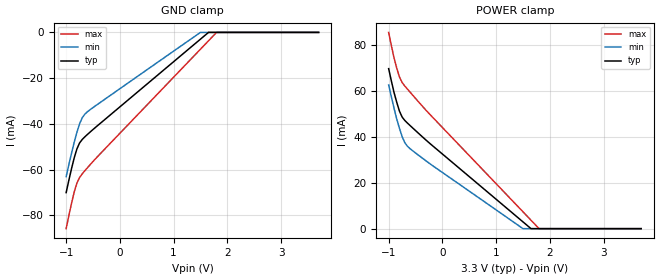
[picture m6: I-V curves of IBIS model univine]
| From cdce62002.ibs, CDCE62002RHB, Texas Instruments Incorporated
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|   Model   univine
[Model]   univine
Model_type   Input
Polarity   Non-Inverting
Vinl   =   1.30
Vinh   =   1.80
|Variable   typ   min   max
C_comp   9.336e-13   4.738e-14   2.334e-12
|Variable   typ   min   max
[Voltage range]   3.3   3.0   3.6
|Variable   typ   min   max
[Temperature range]  25   85   0
[GND_clamp]
|Volts   typ   min   max
-1V       -70.09mA   -63.08mA   -85.83mA
-900mV    -59.59mA   -52.85mA   -74.75mA
-850mV    -54.89mA   -48.07mA   -69.84mA
-800mV    -50.98mA   -43.69mA   -65.93mA
-750mV    -48.35mA   -39.98mA   -63.46mA
-700mV    -46.81mA   -37.31mA   -61.86mA
-650mV    -45.64mA   -35.7mA    -60.45mA
-400mV    -40.48mA   -31.22mA   -53.93mA
1.5V      -2.961mA   0A         -7.354mA
1.65V     0A         0A         -3.677mA
1.8V      0A         0A         0A
3.7V      0A         0A         0A
[POWER_clamp]
|Volts   typ   min   max
-1V       69.73mA    62.62mA    85.53mA
-900mV    59.36mA    52.54mA    74.41mA
-850mV    55.14mA    47.83mA    70.03mA
-800mV    51.28mA    43.84mA    66.17mA
-750mV    48.68mA    40.16mA    63.75mA
-700mV    47.17mA    37.51mA    62.19mA
-650mV    46.01mA    35.9mA     60.81mA
-250mV    37.48mA    28.61mA    50.24mA
1.5V      2.967mA    3.724uA    7.36mA
1.65V     3.26uA     0A         3.684mA
1.8V      0A         0A         3.208uA
3.7V      0A         0A         0A
